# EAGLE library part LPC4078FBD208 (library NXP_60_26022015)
32-bit ARM Cortex-M4 MCU; up to 512 kB flash, 96 kB SRAM; USB Device/Host/OTG; Ethernet; LCD; EMC; SPIFI The LPC408x/7x is an ARM Cortex-M4 based digital signal controller for embedded applications requiring a high level of integration and low power dissipation. The ARM Cortex-M4 is a next generation core that offers system enhancements such as low power consumption, enhanced debug features, and a high level of support block integration. The ARM Cortex-M4 CPU incorporates a 3-stage pipeline, uses a Harvard architecture with separate local instruction and data buses as well as a third bus for peripherals, and includes an internal prefetch unit that supports speculative branching. The ARM Cortex-M4 supports single-cycle digital signal processing and SIMD instructions. A hardware floating-point processor is integrated in the core for several versions of the part. The LPC408x/7x adds a specialized flash memory accelerator to accomplish optimal performance when executing code from flash. The LPC408x/7x is targeted to operate at up to 120 MHz CPU frequency. The peripheral complement of the LPC408x/7x includes up to 512 kB of flash program memory, up to 96 kB of SRAM data memory, up to 4032 byte of EEPROM data memory, External Memory controller (EMC), LCD, Ethernet, USB Device/Host/OTG, an SPI Flash Interface (SPIFI), a General Purpose DMA controller, five UARTs, three SSP controllers, three I 2 C-bus interfaces, a Quadrature Encoder Interface, four general purpose timers, two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
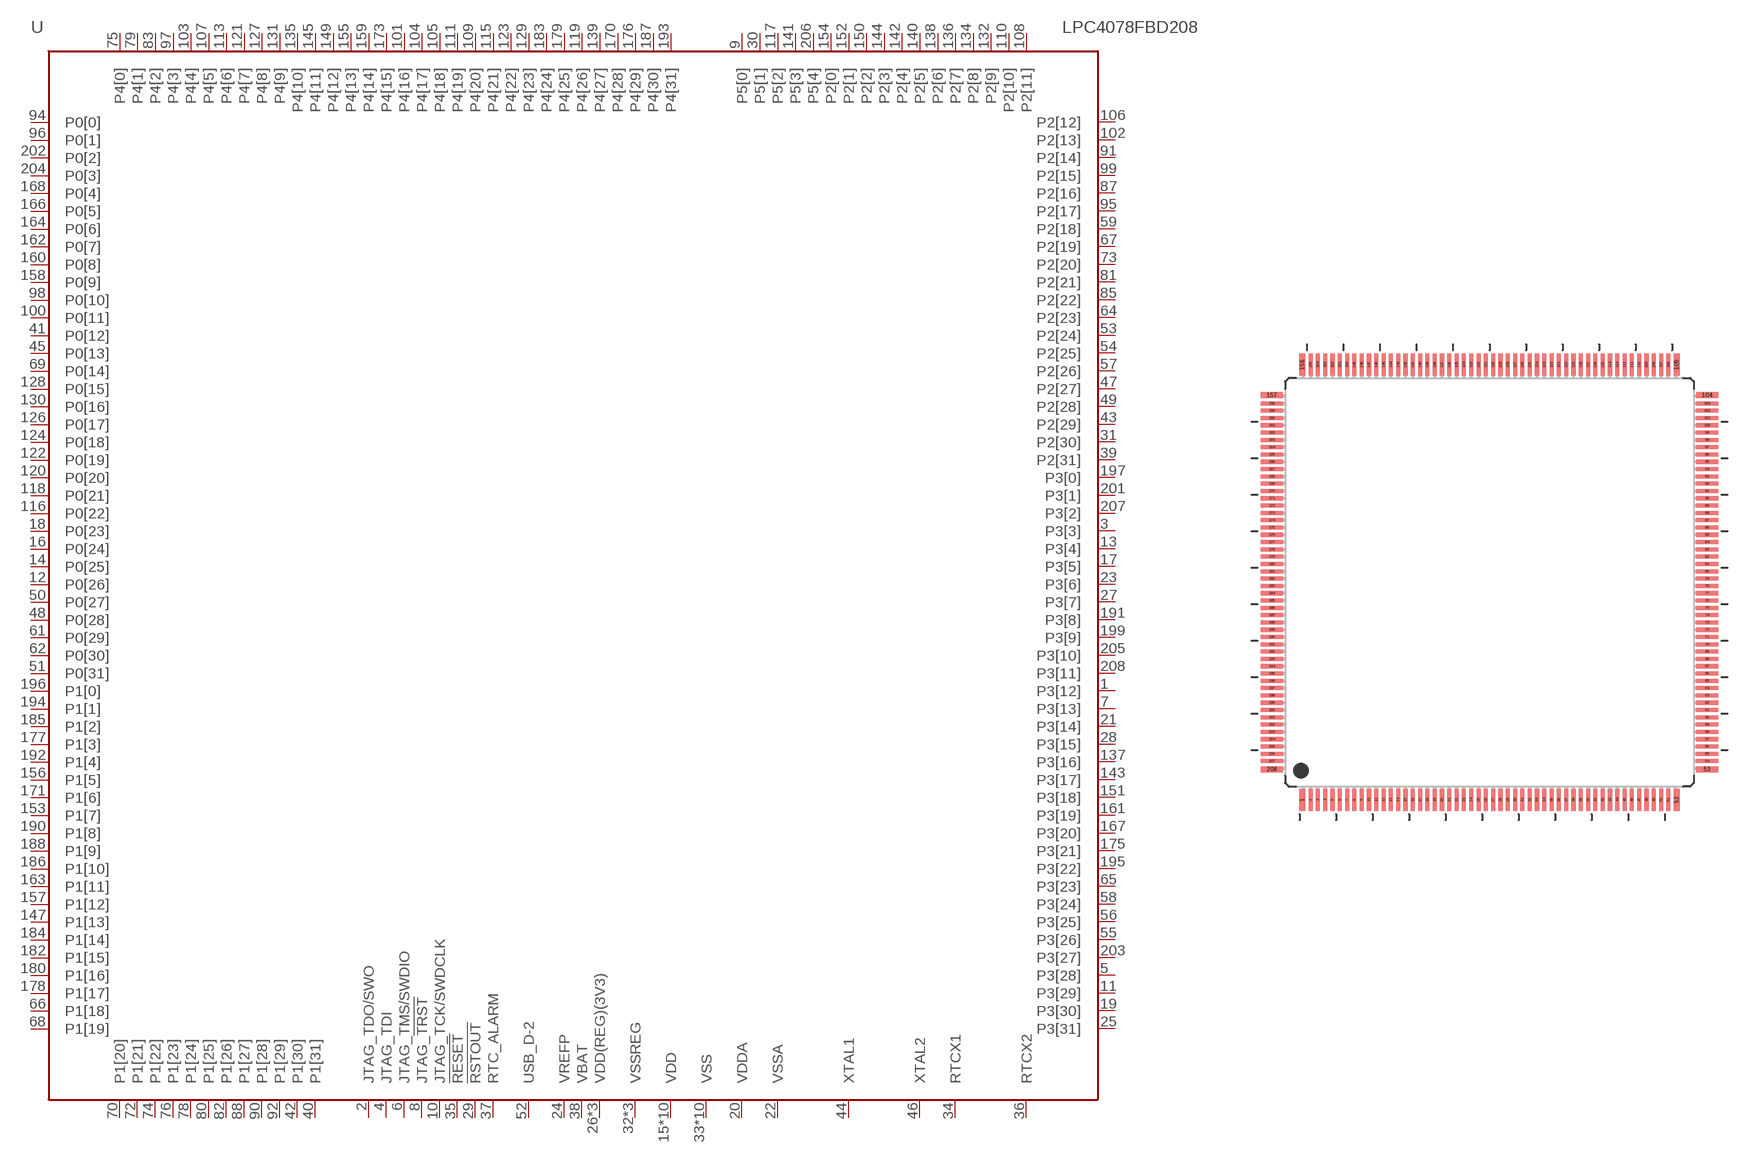
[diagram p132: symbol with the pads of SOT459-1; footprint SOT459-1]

Designator prefix U

## LPC4078FBD208  [SOT459-1]
1  P3[12]
2  JTAG_TDO/SWO  out
3  P3[3]
4  JTAG_TDI  in
5  P3[28]
6  JTAG_TMS/SWDIO  in
7  P3[13]
8  JTAG_!TRST  in
9  P5[0]
10  JTAG_TCK/SWDCLK  in
11  P3[29]
12  P0[26]
13  P3[4]
14  P0[25]
15  VDD  pwr
16  P0[24]
17  P3[5]
18  P0[23]
19  P3[30]
20  VDDA  pwr
21  P3[14]
22  VSSA  pwr
23  P3[6]
24  VREFP  pwr
25  P3[31]
26  VDD(REG)(3V3)  pwr
27  P3[7]
28  P3[15]
29  !RSTOUT!  out
30  P5[1]
31  P2[30]
32  VSSREG  pwr
33  VSS  pwr
34  RTCX1  in
35  !RESET!  in
36  RTCX2  out
37  RTC_ALARM  out
38  VBAT  pwr
39  P2[31]
40  P1[31]
41  P0[12]
42  P1[30]
43  P2[29]
44  XTAL1  in
45  P0[13]
46  XTAL2  out
47  P2[27]
48  P0[28]
49  P2[28]
50  P0[27]
51  P0[31]
52  USB_D-2
53  P2[24]
54  P2[25]
55  P3[26]
56  P3[25]
57  P2[26]
58  P3[24]
59  P2[18]
60  VDD  pwr
61  P0[29]
62  P0[30]
63  VSS  pwr
64  P2[23]
65  P3[23]
66  P1[18]
67  P2[19]
68  P1[19]
69  P0[14]
70  P1[20]
71  VDD  pwr
72  P1[21]
73  P2[20]
74  P1[22]
75  P4[0]
76  P1[23]
77  VSS  pwr
78  P1[24]
79  P4[1]
80  P1[25]
81  P2[21]
82  P1[26]
83  P4[2]
84  VSSREG  pwr
85  P2[22]
86  VDD(REG)(3V3)  pwr
87  P2[16]
88  P1[27]
89  VDD  pwr
90  P1[28]
91  P2[14]
92  P1[29]
93  VSS  pwr
94  P0[0]
95  P2[17]
96  P0[1]
97  P4[3]
98  P0[10]
99  P2[15]
100  P0[11]
101  P4[16]
102  P2[13]
103  P4[4]
104  P4[17]
105  P4[18]
106  P2[12]
107  P4[5]
108  P2[11]
109  P4[20]
110  P2[10]
111  P4[19]
112  VDD  pwr
113  P4[6]
114  VSS  pwr
115  P4[21]
116  P0[22]
117  P5[2]
118  P0[21]
119  P4[26]
120  P0[20]
121  P4[7]
122  P0[19]
123  P4[22]
124  P0[18]
125  VDD  pwr
126  P0[17]
127  P4[8]
128  P0[15]
129  P4[23]
130  P0[16]
131  P4[9]
132  P2[9]
133  VSS  pwr
134  P2[8]
135  P4[10]
136  P2[7]
137  P3[16]
138  P2[6]
139  P4[27]
140  P2[5]
141  P5[3]
142  P2[4]
143  P3[17]
144  P2[3]
145  P4[11]
146  VDD  pwr
147  P1[13]
148  VSS  pwr
149  P4[12]
150  P2[2]
151  P3[18]
152  P2[1]
153  P1[7]
154  P2[0]
155  P4[13]
156  P1[5]
157  P1[12]
158  P0[9]
159  P4[14]
160  P0[8]
161  P3[19]
162  P0[7]
163  P1[11]
164  P0[6]
165  VDD  pwr
166  P0[5]
167  P3[20]
168  P0[4]
169  VSS  pwr
170  P4[28]
171  P1[6]
172  VSSREG  pwr
173  P4[15]
174  VDD(REG)(3V3)  pwr
175  P3[21]
176  P4[29]
177  P1[3]
178  P1[17]
179  P4[25]
180  P1[16]
181  VDD  pwr
182  P1[15]
183  P4[24]
184  P1[14]
185  P1[2]
186  P1[10]
187  P4[30]
188  P1[9]
189  VSS  pwr
190  P1[8]
191  P3[8]
192  P1[4]
193  P4[31]
194  P1[1]
195  P3[22]
196  P1[0]
197  P3[0]
198  VDD  pwr
199  P3[9]
200  VSS  pwr
201  P3[1]
202  P0[2]
203  P3[27]
204  P0[3]
205  P3[10]
206  P5[4]
207  P3[2]
208  P3[11]

## Footprint SOT459-1 (pad centres in mm)
SOT459-1 LQFP208; plastic low profile quad flat package; 208 leads; body 28 x 28 x 1.4 mm JEDEC: MS-026 IEC: 136E30 JEITA: --
smd 0.4 x 1.5: 1 -12.81,-14.9; 52 12.81,-14.9; 105 12.81,14.9; 156 -12.81,14.9
smd 0.28 x 1.5: 2 -12.25,-14.9; 3 -11.75,-14.9; 4 -11.25,-14.9; 5 -10.75,-14.9; 6 -10.25,-14.9; 7 -9.75,-14.9; 8 -9.25,-14.9; 9 -8.75,-14.9; 10 -8.25,-14.9; 11 -7.75,-14.9; 12 -7.25,-14.9; 13 -6.75,-14.9; 14 -6.25,-14.9; 15 -5.75,-14.9; 16 -5.25,-14.9; 17 -4.75,-14.9; 18 -4.25,-14.9; 19 -3.75,-14.9; 20 -3.25,-14.9; 21 -2.75,-14.9; 22 -2.25,-14.9; 23 -1.75,-14.9; 24 -1.25,-14.9; 25 -0.75,-14.9; 26 -0.25,-14.9; 27 0.25,-14.9; 28 0.75,-14.9; 29 1.25,-14.9; 30 1.75,-14.9; 31 2.25,-14.9; 32 2.75,-14.9; 33 3.25,-14.9; 34 3.75,-14.9; 35 4.25,-14.9; 36 4.75,-14.9; 37 5.25,-14.9; 38 5.75,-14.9; 39 6.25,-14.9; 40 6.75,-14.9; 41 7.25,-14.9; 42 7.75,-14.9; 43 8.25,-14.9; 44 8.75,-14.9; 45 9.25,-14.9; 46 9.75,-14.9; 47 10.25,-14.9; 48 10.75,-14.9; 49 11.25,-14.9; 50 11.75,-14.9; 51 12.25,-14.9; 106 12.25,14.9; 107 11.75,14.9; 108 11.25,14.9; 109 10.75,14.9; 110 10.25,14.9; 111 9.75,14.9; 112 9.25,14.9; 113 8.75,14.9; 114 8.25,14.9; 115 7.75,14.9; 116 7.25,14.9; 117 6.75,14.9; 118 6.25,14.9; 119 5.75,14.9; 120 5.25,14.9; 121 4.75,14.9; 122 4.25,14.9; 123 3.75,14.9; 124 3.25,14.9; 125 2.75,14.9; 126 2.25,14.9; 127 1.75,14.9; 128 1.25,14.9; 129 0.75,14.9; 130 0.25,14.9; 131 -0.25,14.9; 132 -0.75,14.9; 133 -1.25,14.9; 134 -1.75,14.9; 135 -2.25,14.9; 136 -2.75,14.9; 137 -3.25,14.9; 138 -3.75,14.9; 139 -4.25,14.9; 140 -4.75,14.9; 141 -5.25,14.9; 142 -5.75,14.9; 143 -6.25,14.9; 144 -6.75,14.9; 145 -7.25,14.9; 146 -7.75,14.9; 147 -8.25,14.9; 148 -8.75,14.9; 149 -9.25,14.9; 150 -9.75,14.9; 151 -10.25,14.9; 152 -10.75,14.9; 153 -11.25,14.9; 154 -11.75,14.9; 155 -12.25,14.9
smd 1.5 x 0.4: 53 14.9,-12.81; 104 14.9,12.81; 157 -14.9,12.81; 208 -14.9,-12.81
smd 1.5 x 0.28: 54 14.9,-12.25; 55 14.9,-11.75; 56 14.9,-11.25; 57 14.9,-10.75; 58 14.9,-10.25; 59 14.9,-9.75; 60 14.9,-9.25; 61 14.9,-8.75; 62 14.9,-8.25; 63 14.9,-7.75; 64 14.9,-7.25; 65 14.9,-6.75; 66 14.9,-6.25; 67 14.9,-5.75; 68 14.9,-5.25; 69 14.9,-4.75; 70 14.9,-4.25; 71 14.9,-3.75; 72 14.9,-3.25; 73 14.9,-2.75; 74 14.9,-2.25; 75 14.9,-1.75; 76 14.9,-1.25; 77 14.9,-0.75; 78 14.9,-0.25; 79 14.9,0.25; 80 14.9,0.75; 81 14.9,1.25; 82 14.9,1.75; 83 14.9,2.25; 84 14.9,2.75; 85 14.9,3.25; 86 14.9,3.75; 87 14.9,4.25; 88 14.9,4.75; 89 14.9,5.25; 90 14.9,5.75; 91 14.9,6.25; 92 14.9,6.75; 93 14.9,7.25; 94 14.9,7.75; 95 14.9,8.25; 96 14.9,8.75; 97 14.9,9.25; 98 14.9,9.75; 99 14.9,10.25; 100 14.9,10.75; 101 14.9,11.25; 102 14.9,11.75; 103 14.9,12.25; 158 -14.9,12.25; 159 -14.9,11.75; 160 -14.9,11.25; 161 -14.9,10.75; 162 -14.9,10.25; 163 -14.9,9.75; 164 -14.9,9.25; 165 -14.9,8.75; 166 -14.9,8.25; 167 -14.9,7.75; 168 -14.9,7.25; 169 -14.9,6.75; 170 -14.9,6.25; 171 -14.9,5.75; 172 -14.9,5.25; 173 -14.9,4.75; 174 -14.9,4.25; 175 -14.9,3.75; 176 -14.9,3.25; 177 -14.9,2.75; 178 -14.9,2.25; 179 -14.9,1.75; 180 -14.9,1.25; 181 -14.9,0.75; 182 -14.9,0.25; 183 -14.9,-0.25; 184 -14.9,-0.75; 185 -14.9,-1.25; 186 -14.9,-1.75; 187 -14.9,-2.25; 188 -14.9,-2.75; 189 -14.9,-3.25; 190 -14.9,-3.75; 191 -14.9,-4.25; 192 -14.9,-4.75; 193 -14.9,-5.25; 194 -14.9,-5.75; 195 -14.9,-6.25; 196 -14.9,-6.75; 197 -14.9,-7.25; 198 -14.9,-7.75; 199 -14.9,-8.25; 200 -14.9,-8.75; 201 -14.9,-9.25; 202 -14.9,-9.75; 203 -14.9,-10.25; 204 -14.9,-10.75; 205 -14.9,-11.25; 206 -14.9,-11.75; 207 -14.9,-12.25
